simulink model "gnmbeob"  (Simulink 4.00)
settings: Solver=ode45  StartTime=0.0  StopTime=Tstop  MaxStep=step_max  RelTol=1e-3
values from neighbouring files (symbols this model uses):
  beob = estim(sys,l,1,1)    [gnmbeobl_i.m]    (also in gnmbeobregl_i.m = estim(sysbeob,l,1,1); gnmbeobregs_i.m = ss(beob.a,beob.b,beob.c,beob.d); gnmbeobreg_i.m = ss([],[0 0],[],0); gnmbeobs_i.m = ss(beob.a,beob.b,beob.c,beob.d))
  beobx0 = [ 0 ]    [gnmbeobreg_i.m]    (also in gnmbeob_i.m)
  CE = 2*pi*CM    (= 240.017678734)    [gnm_i.m]
  CM = 38.2    [gnm_i.m]
  J = 0.012    [gnm_i.m]
  MW = 10    [gnmbeobreg_i.m]    (also in gnmbeob_i.m; gnmregn_i.m = 100; gnm_i.m = 0; lsg_gnmregnss_ini.m = 100)
  PsiN = 0.04    [gnm_i.m]
  RA = 0.250    (= 0.25)    [gnm_i.m]
  T_MW = 0.4    [gnmbeobreg_i.m]    (also in gnmbeob_i.m; gnmregn_i.m = 0.1; gnm_i.m = 0; lsg_gnmregnss_ini.m = 0.1)
  T_t = 0.0001    [gnmbeobreg_i.m]    (also in gnmbeob_i.m; gnmregi_i.m)
  TA = LA / RA    (= 0.016)    [gnm_i.m]
libraries: simulink3 x1

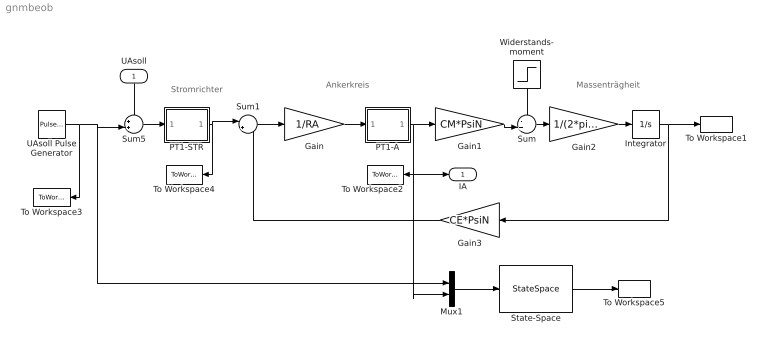
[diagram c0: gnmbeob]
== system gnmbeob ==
  note: Massenträgheit
  note: Ankerkreis
  note: Stromrichter
  UAsoll : Inport  Orientation=down  Port=1  PortDimensions=1
  Gain : Gain  Gain=1/RA  Multiplication=Element-wise(K.*u)  SaturateOnIntegerOverflow=on
  Gain1 : Gain  Gain=CM*PsiN  Multiplication=Element-wise(K.*u)  SaturateOnIntegerOverflow=on
  Gain2 : Gain  Gain=1/(2*pi*J)  Multiplication=Element-wise(K.*u)  SaturateOnIntegerOverflow=on
  Gain3 : Gain  Orientation=left  Gain=CE*PsiN  Multiplication=Element-wise(K.*u)  SaturateOnIntegerOverflow=on
  Integrator : Integrator  ExternalReset=none  InitialConditionSource=internal  InitialCondition=0  LimitOutput=off  UpperSaturationLimit=inf  LowerSaturationLimit=-inf  ShowSaturationPort=off  ShowStatePort=off  AbsoluteTolerance=auto
  Mux1 : Mux  Inputs=2
  PT1-A : Subsystem  mask(PT1){T=TA}
      mask prompts: T "Zeitkonstante"
      mask help: PT1 mit rückgekoppeltem Integrierer
  PT1-STR : Subsystem  mask(PT1){T=T_t}
      mask prompts: T "Zeitkonstante"
      mask help: PT1 mit rückgekoppeltem Integrierer
  State-Space : StateSpace  A=beob.a  B=beob.b  C=beob.c  D=beob.d  X0=beobx0  Realization=auto  AbsoluteTolerance=auto
  Sum : Sum  Inputs=-+|  SaturateOnIntegerOverflow=on
  Sum1 : Sum  Inputs=|+-  SaturateOnIntegerOverflow=on
  Sum5 : Sum  Inputs=++|  SaturateOnIntegerOverflow=on
  To Workspace1 : ToWorkspace  VariableName=N  SampleTime=-1  SaveFormat=Array
  To Workspace2 : ToWorkspace  VariableName=IA  SampleTime=-1  SaveFormat=Array
  To Workspace3 : ToWorkspace  VariableName=UAsoll  SampleTime=-1  SaveFormat=Array
  To Workspace4 : ToWorkspace  VariableName=UA  SampleTime=-1  SaveFormat=Array
  To Workspace5 : ToWorkspace  VariableName=ybeob  SampleTime=-1  SaveFormat=Array
  UAsoll Pulse Generator : simulink3/Sources/Pulse Generator  period=T_UAsoll  duty=50  amplitude=UA_soll  start=0
  Widerstands- moment : Step  Orientation=down  Time=T_MW  Before=0  After=MW  SampleTime=0
  IA : Outport  Port=1
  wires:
  Gain/1 -> PT1-A/1(In1)
  Gain1/1 -> Sum/2
  Sum/1 -> Gain2/1
  Gain2/1 -> Integrator/1
  Integrator/1 -> To Workspace1/1, Gain3/1
  PT1-A/1(Out1) -> Gain1/1, IA/1, To Workspace2/1, Mux1/2
  Sum1/1 -> Gain/1
  UAsoll/1 -> Sum5/1
  Sum5/1 -> PT1-STR/1(In1)
  Widerstands- moment/1 -> Sum/1
  Gain3/1 -> Sum1/2
  Mux1/1 -> State-Space/1
  State-Space/1 -> To Workspace5/1
  PT1-STR/1(Out1) -> Sum1/1, To Workspace4/1
  UAsoll Pulse Generator/1 -> To Workspace3/1, Sum5/2, Mux1/1

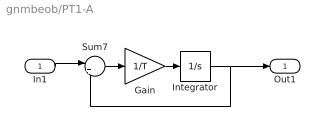
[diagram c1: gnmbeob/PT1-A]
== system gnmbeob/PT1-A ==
  In1 : Inport  Port=1
  Gain : Gain  Gain=1/T  Multiplication=Element-wise(K.*u)  SaturateOnIntegerOverflow=on
  Integrator : Integrator  ExternalReset=none  InitialConditionSource=internal  InitialCondition=0  LimitOutput=off  UpperSaturationLimit=inf  LowerSaturationLimit=-inf  ShowSaturationPort=off  ShowStatePort=off  AbsoluteTolerance=auto
  Sum7 : Sum  Inputs=|+-  SaturateOnIntegerOverflow=on
  Out1 : Outport  Port=1
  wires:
  Integrator/1 -> Sum7/2, Out1/1
  Gain/1 -> Integrator/1
  Sum7/1 -> Gain/1
  In1/1 -> Sum7/1

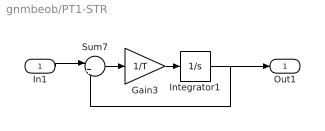
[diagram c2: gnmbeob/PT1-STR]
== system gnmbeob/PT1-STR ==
  In1 : Inport  Port=1
  Gain3 : Gain  Gain=1/T  Multiplication=Element-wise(K.*u)  SaturateOnIntegerOverflow=on
  Integrator1 : Integrator  ExternalReset=none  InitialConditionSource=internal  InitialCondition=0  LimitOutput=off  UpperSaturationLimit=inf  LowerSaturationLimit=-inf  ShowSaturationPort=off  ShowStatePort=off  AbsoluteTolerance=auto
  Sum7 : Sum  Inputs=|+-  SaturateOnIntegerOverflow=on
  Out1 : Outport  Port=1
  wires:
  Integrator1/1 -> Sum7/2, Out1/1
  Gain3/1 -> Integrator1/1
  Sum7/1 -> Gain3/1
  In1/1 -> Sum7/1
